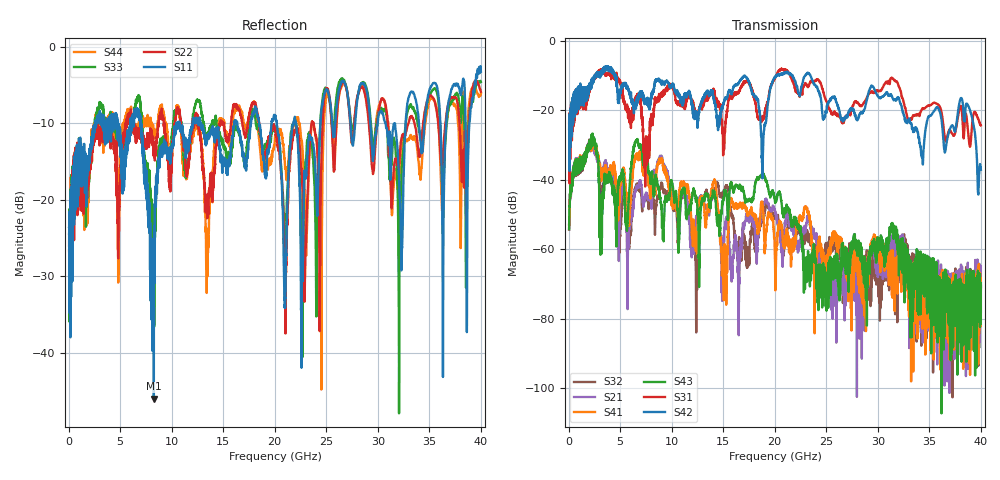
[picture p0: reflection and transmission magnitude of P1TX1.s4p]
!Agilent Technologies,N5245A,MY49151084,A.09.20.08
!Agilent N5245A: A.09.20.08
!Date: Thursday, March 01, 2012 14:28:51
!Correction: S11(Full 4 Port(1,2,3,4))
!S12(Full 4 Port(1,2,3,4))
!S13(Full 4 Port(1,2,3,4))
!S14(Full 4 Port(1,2,3,4))
!S21(Full 4 Port(1,2,3,4))
!S22(Full 4 Port(1,2,3,4))
!S23(Full 4 Port(1,2,3,4))
!S24(Full 4 Port(1,2,3,4))
!S31(Full 4 Port(1,2,3,4))
!S32(Full 4 Port(1,2,3,4))
!S33(Full 4 Port(1,2,3,4))
!S34(Full 4 Port(1,2,3,4))
!S41(Full 4 Port(1,2,3,4))
!S42(Full 4 Port(1,2,3,4))
!S43(Full 4 Port(1,2,3,4))
!S44(Full 4 Port(1,2,3,4))
!S4P File: Measurements: <S11,S12,S13,S14>,
!<S21,S22,S23,S24>,
!<S31,S32,S33,S34>,
!<S41,S42,S43,S44>:
# Hz S  dB  R 50
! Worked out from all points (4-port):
!   3996 points, 50 MHz to 40 GHz, reference 50 ohm
!   strongest paths, dB at 50 MHz, 10.04 GHz, 20.03 GHz, 30.02 GHz, 40 GHz:
!     S42: -25.4, -12.8, -10.4, -16.0, -37.1
!     S31: -23.7, -13.5, -10.8, -14.5, -24.3
!     S43: -54.2, -41.0, -46.2, -56.6, -69.7
!     S41: -53.0, -46.7, -63.6, -59.7, -70.4
!     S21: -52.7, -43.7, -49.2, -61.8, -78.1
!     S32: -54.4, -46.7, -49.8, -67.7, -70.9
!   lowest |S11| = -46.0 dB at 8.27 GHz (marker M1), VSWR 1.01, Z = 49.8 - j0.477 ohm
!   |S11| at or under -10 dB: start of sweep to 2.585 GHz; 7.014 GHz to 10.48 GHz (3.463 GHz wide, 39.6 % of centre); 12.79 GHz to 16.07 GHz (3.276 GHz wide, 22.7 % of centre)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
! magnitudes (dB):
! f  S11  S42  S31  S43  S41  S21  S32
! 50 MHz  -23.5  -25.4  -23.7  -54.2  -53.0  -52.7  -54.4
! 2.34 GHz  -11.2  -12.3  -11.9  -27.1  -28.1  -29.2  -27.4
! 5.79 GHz  -11.4  -13.8  -21.0  -47.8  -50.9  -59.5  -57.6
! 8.27 GHz  -46.0  -14.0  -19.4  -44.9  -41.3  -37.1  -46.1
! 16.47 GHz  -10.9  -12.3  -15.1  -42.1  -47.2  -74.6  -62.2
! 38.07 GHz  -6.4  -16.5  -18.8  -72.5  -82.4  -64.4  -72.1
! 40 GHz  -3.3  -37.1  -24.3  -69.7  -70.4  -78.1  -70.9
